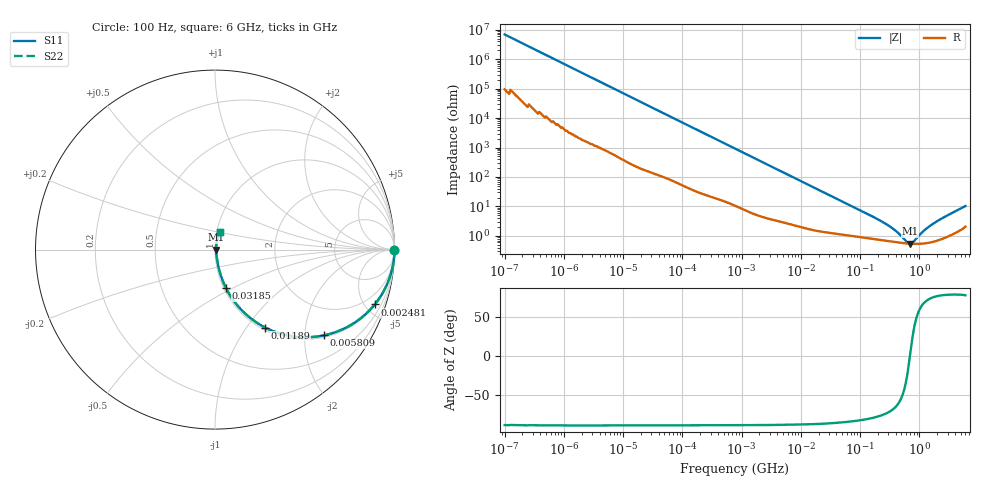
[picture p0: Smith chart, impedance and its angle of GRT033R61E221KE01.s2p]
!Murata Part Number: GRT033R61E221KE01
!These Parameters are Measured in Series Mode Connection
!Data Generated on Jun 19, 2026
!  o--ll--o
!Port1  Port2
!  o------o
!Operation Temp=25[degC], DC Bias Voltage=0[V]
!Freq. Start=100[Hz] Stop=6[GHz] 401[Steps]
# Hz S RI R 50
!Freq.(Hz) S11(Real) S11(Imag) S21(Real) S21(Imag) S12(Real) S12(Imag) S22(Real) S22(Imag)
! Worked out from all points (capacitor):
!   401 points, 100 Hz to 6 GHz, reference 50 ohm
!   read as one part in series: C = 230 pF near 109 Hz
!   lowest |Z| = 545 mohm at 699.5 MHz (marker M1)
!   series resonance near 694.5 MHz, so ESL is about 230 pH
!   S11 on the Smith chart (normalised r, x): 100 Hz: open; 2.481 MHz: 1.08, -5.80; 5.809 MHz: 1.05, -2.49; 11.89 MHz: 1.04, -1.23; 31.85 MHz: 1.03, -0.46; 6 GHz: 1.04, +0.20
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100  1 -1.45e-05  2e-07 1.45e-05  2e-07 1.45e-05  1 -1.45e-05
686  1 -9.88e-05  7e-07 9.88e-05  7e-07 9.88e-05  1 -9.88e-05
2008  1 -0.000288  1.6e-06 0.000288  1.6e-06 0.000288  1 -0.000288
40335  0.9999 -0.00573  7.02e-05 0.00573  7.02e-05 0.00573  0.9999 -0.00573
241822  0.9985 -0.0341  0.00145 0.0341  0.00145 0.0341  0.9985 -0.0341
774597  0.9872 -0.1069  0.0128 0.1069  0.0128 0.1069  0.9872 -0.1069
2481164  0.8903 -0.3055  0.1097 0.3055  0.1097 0.3055  0.8903 -0.3055
3712478  0.7866 -0.4011  0.2134 0.4011  0.2134 0.4011  0.7866 -0.4011
5809218  0.6065 -0.4779  0.3935 0.4779  0.3935 0.4779  0.6065 -0.4779
8311524  0.4354 -0.4834  0.5646 0.4834  0.5646 0.4834  0.4354 -0.4834
1.189169e7  0.2797 -0.4343  0.7203 0.4343  0.7203 0.4343  0.2797 -0.4343
1.555665e7  0.1895 -0.3753  0.8105 0.3753  0.8105 0.3753  0.1895 -0.3753
3.184506e7  0.0615 -0.2145  0.9385 0.2145  0.9385 0.2145  0.0615 -0.2145
8.154455e7  0.0177 -0.089  0.9823 0.089  0.9823 0.089  0.0177 -0.089
3.124326e8  0.00702 -0.0202  0.993 0.0202  0.993 0.0202  0.00702 -0.0202
4.274388e8  0.00617 -0.0118  0.9938 0.0118  0.9938 0.0118  0.00617 -0.0118
6.11557e8  0.00554 -0.00304  0.9945 0.00304  0.9945 0.00304  0.00554 -0.00304
6.994765e8  0.00542 0.000173  0.9946 -0.000173  0.9946 -0.000173  0.00542 0.000173
8.000355e8  0.00536 0.00342  0.9946 -0.00342  0.9946 -0.00342  0.00536 0.00342
1.197065e9  0.00571 0.0139  0.9943 -0.0139  0.9943 -0.0139  0.00571 0.0139
1.712697e9  0.00691 0.0249  0.9931 -0.0249  0.9931 -0.0249  0.00691 0.0249
6e9  0.0298 0.0965  0.9702 -0.0965  0.9702 -0.0965  0.0298 0.0965
